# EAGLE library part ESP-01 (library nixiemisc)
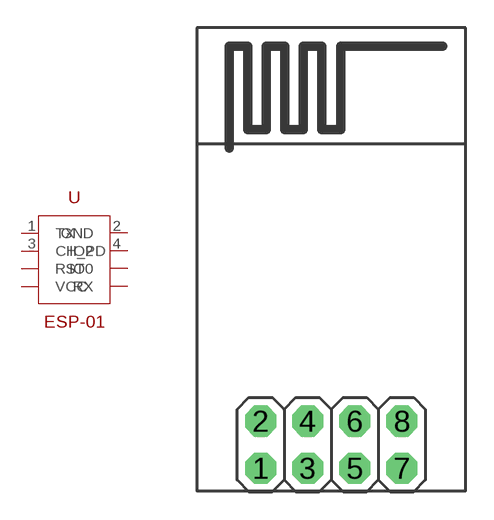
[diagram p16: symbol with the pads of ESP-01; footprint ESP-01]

Designator prefix U

## ESP-01  [ESP-01]
1  TX
2  GND  pwr
3  CH_PD  pas
4  IO2
5  RST  pas
6  IO0
7  VCC  pwr
8  RX

## Footprint ESP-01 (pad centres in mm)
PIN HEADER
drill 1.016 pad 1.676 octagon: 1 -3.81,-1.27; 2 -3.81,1.27; 3 -1.27,-1.27; 4 -1.27,1.27; 5 1.27,-1.27; 6 1.27,1.27; 7 3.81,-1.27; 8 3.81,1.27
